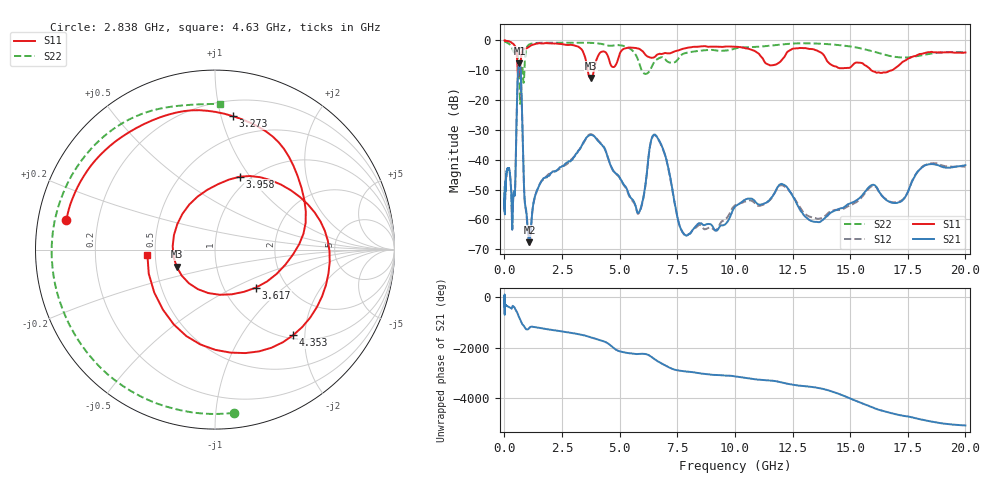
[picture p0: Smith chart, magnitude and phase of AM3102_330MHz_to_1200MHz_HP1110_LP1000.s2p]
! Date/Time: Tue, Sep 11, 2018 5:23 PM
! Network Analyzer: Agilent Technologies E8362B Rev: A.07.50.63
! Sweep from 0.010 to 20.000 GHz, 1601 Points, Sweep Type: LOG
! Power Supply: 4.949 V, 0.001 A
# Hz S DB R 50
!freq MagS11 AngS11 MagS21 AngS21 MagS12 AngS12 MagS22 AngS22
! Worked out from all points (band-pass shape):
!   1601 points, 10 MHz to 20 GHz, reference 50 ohm
!   highest |S21| = -7.69 dB at 650.9 MHz (marker M1); lowest = -67.6 dB at 1.087 GHz (marker M2)
!   |S21| within 3 dB of the highest: 590.7 MHz to 706.1 MHz (115.4 MHz wide, 17.8 % of centre)
!   lowest |S11| = -12.6 dB at 3.757 GHz (marker M3), VSWR 1.61, Z = 31.9 - j6.47 ohm
!   |S11| at or under -10 dB: 573.1 MHz to 634.9 MHz (61.72 MHz wide, 10.2 % of centre); 3.614 GHz to 3.888 GHz (274 MHz wide, 7.31 % of centre); 15.91 GHz to 16.81 GHz (896.1 MHz wide, 5.48 % of centre)
!   |S22| runs from -21.3 to -0.3 dB; largest |S21 - S12| = 0.0055
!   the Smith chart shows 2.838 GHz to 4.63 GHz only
!   S11 on the Smith chart (normalised r, x): 2.838 GHz: 0.09, +0.10; 3.273 GHz: 0.32, +1.09; 3.617 GHz: 1.41, -0.66; 3.958 GHz: 0.90, +0.89; 4.353 GHz: 1.07, -1.75; 4.63 GHz: 0.45, -0.03
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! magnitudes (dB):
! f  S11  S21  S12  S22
! 10 MHz  0.0  -49.2  -54.2  -0.3
! 35.55 MHz  -0.1  -51.6  -52.0  -0.4
! 126.4 MHz  -0.2  -43.3  -43.1  -0.8
! 249.3 MHz  -0.5  -45.5  -45.3  -1.4
! 339.5 MHz  -1.0  -63.5  -63.0  -2.6
! 447.2 MHz  -1.8  -52.0  -51.9  -3.9
! 650.9 MHz  -9.5  -7.7  -7.7  -14.0
! 729.5 MHz  -5.4  -14.6  -14.6  -11.9
! 873.8 MHz  -2.8  -52.7  -53.0  -9.2
! 1.087 GHz  -2.0  -67.6  -68.7  -1.3
! 1.59 GHz  -1.0  -47.4  -47.3  -0.8
! 2.838 GHz  -1.5  -40.6  -40.4  -0.8
! 3.273 GHz  -2.5  -36.5  -36.3  -0.8
! 3.617 GHz  -10.1  -32.2  -32.0  -0.8
! 3.757 GHz  -12.6  -31.6  -31.5  -0.8
! 3.958 GHz  -7.4  -32.7  -32.5  -0.9
! 4.353 GHz  -3.8  -36.4  -36.2  -1.5
! 4.63 GHz  -8.5  -42.2  -42.3  -1.8
! 5.652 GHz  -2.5  -54.6  -54.8  -4.3
! 6.549 GHz  -5.4  -31.6  -31.8  -6.8
! 7.92 GHz  -2.5  -65.4  -65.2  -4.1
! 20 GHz  -4.1  -41.8  -42.3  -4.0
